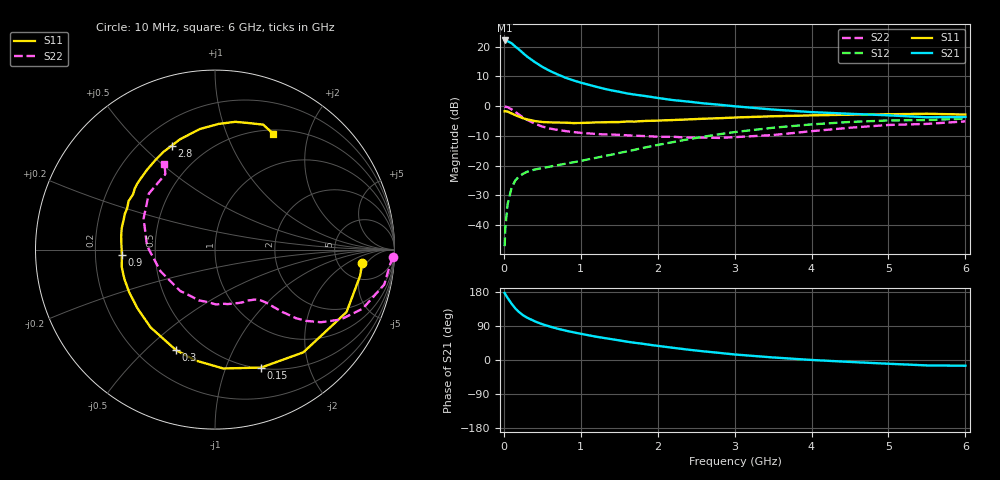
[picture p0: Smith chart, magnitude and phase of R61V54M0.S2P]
! SIEMENS Small Signal Semiconductors
! BFR193
! Si NPN RF Bipolar Junction Transistor in SOT23
! VCE = 1.5 V  IC = 4 mA
! Common Emitter S-Parameters:  May  1996
# GHz  S  MA  R  50
!  f  S11  S21  S12  S22
! GHz  MAG  ANG  MAG  ANG  MAG  ANG  MAG  ANG
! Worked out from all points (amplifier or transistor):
!   36 points, 10 MHz to 6 GHz, reference 50 ohm
!   highest |S21| = 22.1 dB at 10 MHz (marker M1)
!   |S21| within 3 dB of that: start of sweep to 195.6 MHz
!   unconditionally stable (mu >= 1): 931.3 MHz to 2.069 GHz
!   at 250 MHz: K = 0.37, MSG = 20.3 dB, |S12| = -22.8 dB
!   at 1.4 GHz: K = 1.08, MAG = 9.1 dB, |S12| = -16.3 dB
!   at 6 GHz: K = 0.99, MSG = 0.3 dB, |S12| = -4.2 dB
!   S11 on the Smith chart (normalised r, x): 10 MHz: 8.41, -3.96; 150 MHz: 0.51, -1.34; 300 MHz: 0.36, -0.62; 900 MHz: 0.32, -0.03; 2.8 GHz: 0.32, +0.62; 6 GHz: 0.55, +1.48
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0.01  0.823 -5.3  12.79 176.9  0.0044 84.3  0.9927 -2.4
0.02  0.8216 -10.2  12.54 173.2  0.0092 85.8  0.9799 -4.7
0.05  0.8113 -25.4  12.42 163.6  0.0227 77.3  0.9627 -11.7
0.1  0.7549 -49.3  11.5 148.7  0.0421 66.7  0.8862 -21.8
0.15  0.7058 -68.6  10.07 135.9  0.0565 57.8  0.8011 -29.1
0.2  0.6641 -86.0  8.961 126.0  0.0661 52.3  0.7162 -34.4
0.25  0.6272 -100.0  7.826 118.0  0.0727 47.9  0.6435 -38.1
0.3  0.6007 -111.2  6.881 112.0  0.0786 45.6  0.5904 -40.3
0.4  0.5627 -129.6  5.568 102.3  0.0858 42.7  0.5102 -42.8
0.5  0.5419 -143.0  4.595 94.4  0.091 42.3  0.4539 -44.5
0.6  0.5338 -153.7  3.921 88.2  0.0961 43.2  0.4196 -45.6
0.7  0.5308 -162.2  3.422 82.5  0.1017 44.2  0.3987 -46.7
0.9  0.5199 -176.5  2.731 73.3  0.1136 47.3  0.3673 -49.5
1.1  0.5275 172.2  2.302 65.3  0.1277 50.9  0.3483 -53.7
1.3  0.5348 162.7  1.973 58.2  0.1442 53.5  0.335 -58.2
1.6  0.5523 150.7  1.642 48.4  0.1733 56.0  0.324 -66.9
2.2  0.5847 130.1  1.268 32.2  0.2487 55.7  0.3057 -88.9
2.8  0.6273 112.6  1.059 18.8  0.3368 49.5  0.2924 -119.0
3.5  0.6773 97.1  0.878 6.7  0.4339 38.4  0.3269 -158.4
4.5  0.7208 81.0  0.745 -5.1  0.5429 20.9  0.434 156.4
5.5  0.7462 68.9  0.651 -14.3  0.5842 3.8  0.5034 123.3
6  0.7227 63.4  0.659 -15.2  0.619 -1.1  0.5554 120.5
